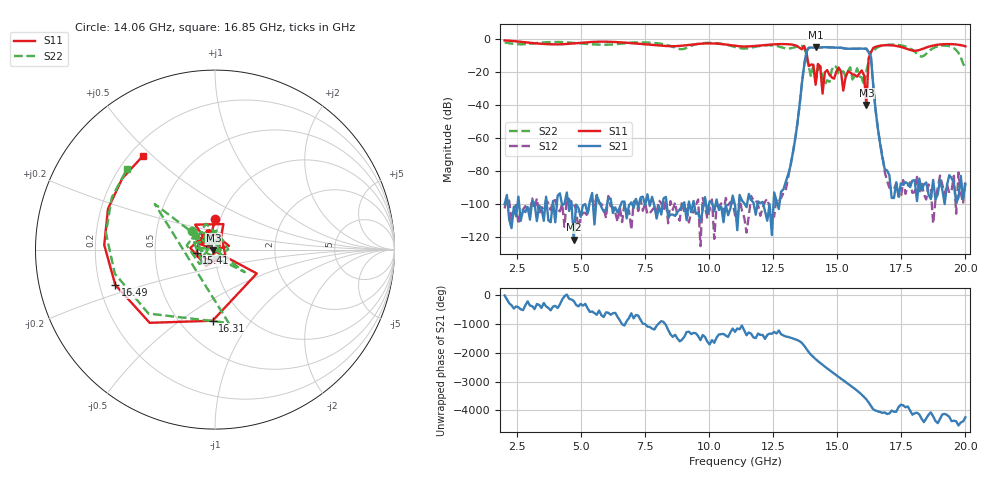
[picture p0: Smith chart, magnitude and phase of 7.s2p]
!Keysight Technologies,N5234A,MY52241180,A.10.60.03
!Date: Friday, January 20, 2023 09:34:39
!Correction: S11(Full 2 Port(1,2))
!S21(Full 2 Port(1,2))
!S12(Full 2 Port(1,2))
!S22(Full 2 Port(1,2))
!S2P File: Measurements: S11, S21, S12, S22:
# Hz S  dB  R 50
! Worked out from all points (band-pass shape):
!   201 points, 2 GHz to 20 GHz, reference 50 ohm
!   highest |S21| = -4.80 dB at 14.15 GHz (marker M1); lowest = -122.0 dB at 4.7 GHz (marker M2)
!   |S21| within 3 dB of the highest: 13.79 GHz to 16.22 GHz (2.434 GHz wide, 16.2 % of centre)
!   lowest |S11| = -40.0 dB at 16.13 GHz (marker M3), VSWR 1.02, Z = 49.1 - j0.374 ohm
!   |S11| at or under -10 dB: 13.81 GHz to 16.26 GHz (2.444 GHz wide, 16.3 % of centre)
!   |S22| runs from -28.1 to -1.7 dB; largest |S21 - S12| = 0.00066
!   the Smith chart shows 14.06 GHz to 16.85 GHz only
!   S11 on the Smith chart (normalised r, x): 14.06 GHz: 0.94, +0.33; 15.41 GHz: 0.81, -0.03; 16.31 GHz: 0.71, -0.67; 16.49 GHz: 0.27, -0.16; 16.85 GHz: 0.25, +0.47
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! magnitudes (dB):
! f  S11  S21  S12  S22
! 2 GHz  -0.7  -100.4  -102.9  -1.9
! 4.7 GHz  -2.5  -122.0  -100.0  -2.2
! 5.06 GHz  -2.0  -101.0  -105.5  -2.7
! 8.03 GHz  -3.8  -101.5  -98.0  -2.6
! 11 GHz  -4.0  -100.8  -107.0  -4.7
! 13.07 GHz  -3.0  -82.5  -84.5  -5.6
! 13.79 GHz  -7.7  -7.4  -7.4  -10.3
! 14.06 GHz  -15.5  -5.1  -5.1  -15.7
! 14.15 GHz  -27.6  -4.8  -4.8  -26.2
! 14.24 GHz  -15.0  -4.9  -4.9  -18.2
! 14.42 GHz  -33.1  -4.9  -4.9  -22.6
! 14.6 GHz  -18.8  -4.9  -4.9  -25.0
! 15.23 GHz  -31.3  -5.4  -5.4  -19.5
! 15.41 GHz  -19.7  -5.8  -5.8  -19.3
! 15.95 GHz  -19.0  -5.6  -5.6  -23.3
! 16.13 GHz  -40.0  -5.7  -5.7  -19.6
! 16.22 GHz  -11.4  -7.8  -7.8  -13.6
! 16.31 GHz  -8.0  -10.6  -10.6  -7.5
! 16.49 GHz  -4.6  -43.0  -42.9  -5.8
! 16.85 GHz  -3.6  -79.0  -80.7  -3.6
! 17.03 GHz  -3.6  -82.6  -90.3  -3.3
! 20 GHz  -4.3  -88.2  -85.1  -17.3
